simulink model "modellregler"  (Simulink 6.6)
settings: Solver=ode45  StartTime=0.0  StopTime=10.0  FixedStep=0.01  RelTol=1e-3
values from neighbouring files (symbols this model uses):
  Aa = [-0.1420]    [regler.m]
  Bb = [0.3420]    [regler.m]
  Cc = [0.4158]    [regler.m]
  stoergroesse = ausgang_ein/8    [regler.m]
libraries: simulink_extras x1

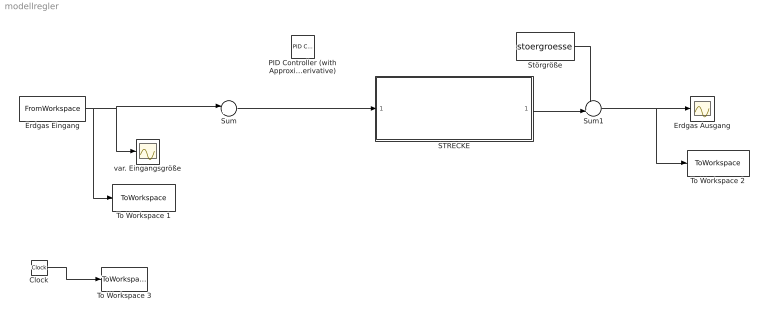
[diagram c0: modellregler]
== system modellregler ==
  Clock : Clock
  Erdgas Ausgang : Scope
  Erdgas Eingang : FromWorkspace  VariableName=eingang_ein  SampleTime=0
  PID Controller (with Approximate Derivative) : simulink_extras/Additional Linear/PID Controller (with Approximate Derivative)  SystemSampleTime=-1  P=0  I=0  D=250  N=10
  STRECKE : Subsystem
  Störgröße : Constant  Value=stoergroesse
  Sum : Sum  Inputs=|+-
  Sum1 : Sum  Inputs=-+|
  To Workspace 1 : ToWorkspace  VariableName=eingang_aus  SampleTime=-1  SaveFormat=Array
  To Workspace 2 : ToWorkspace  VariableName=ausgang_aus  SampleTime=-1  SaveFormat=Array
  To Workspace 3 : ToWorkspace  VariableName=zeit  SampleTime=-1  SaveFormat=Array
  var. Eingangsgröße : Scope
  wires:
  Clock/1 -> To Workspace 3/1
  Erdgas Eingang/1 -> To Workspace 1/1, var. Eingangsgröße/1, Sum/1
  Sum1/1 -> Erdgas Ausgang/1, To Workspace 2/1
  STRECKE/1(ausgang) -> Sum1/2
  Störgröße/1 -> Sum1/1
  Sum/1 -> STRECKE/1(eingang)

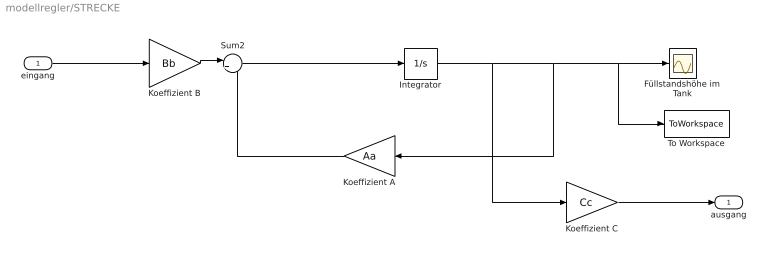
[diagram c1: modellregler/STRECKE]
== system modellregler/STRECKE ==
  eingang : Inport
  Füllstandshöhe im Tank : Scope
  Integrator : Integrator
  Koeffizient A : Gain  Orientation=left  Gain=Aa
  Koeffizient B : Gain  Gain=Bb
  Koeffizient C : Gain  Gain=Cc
  Sum2 : Sum  Inputs=|++
  To Workspace : ToWorkspace  VariableName=fuellhoehe_2  SampleTime=-1  SaveFormat=Array
  ausgang : Outport
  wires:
  Sum2/1 -> Integrator/1
  Integrator/1 -> Füllstandshöhe im Tank/1, To Workspace/1, Koeffizient A/1, Koeffizient C/1
  Koeffizient B/1 -> Sum2/1
  Koeffizient A/1 -> Sum2/2
  Koeffizient C/1 -> ausgang/1
  eingang/1 -> Koeffizient B/1
